| TEXAS INSTRUMENTS INCORPORATED
| Standard Linear and Logic Group
| IBIS Model of SN74LVCH16T245
| 16-Bit Dual-Supply Bus Transceiver With Configurable Voltage
| Translation and 3-State Outputs
| This file contains package information for the following:
|  TSSOP 48-pin (DGG) package as [Component] LVCH16T245_DGG
|  TVSOP 48-pin (DGV) package as [Component] LVCH16T245_DGV
|  VFBGA 48-pin (GQL) package as [Component] LVCH16T245_GQL
|  VFBGA 48-pin (ZQL) package as [Component] LVCH16T245_ZQL
| This device can be powered at the following Vccs:
|  1.8 volt Vcc
|  2.5 volt Vcc
|  3.3 volt Vcc
|  5 volt Vcc
| This file provides unique models under the [Model Selector] for each Vcc.
| For operation at a specific Vcc, select the appropriate model after each
| [Model Selector] keyword.
[IBIS Ver]   3.2
[Comment char]  |_char
[File Name]   sn74lvch16t245.ibs
[File Rev]   1.1 | x_die
[Date]   October 04, 2005
[Source]   Data created from TI-SPICE simulations at TI-SLL.
[Notes]   The following is an IBIS list for the LVCH16T245.
   Please contact sllibis@ti.com with questions and
   comments concerning SLL IBIS models.
   - FILE REV HISTORY
   - 1.1 Release IBIS file on 09/20/05
   - Power-clamp data has been deleted since there is no
   power-clamp diode in the device.
   - Due to presence of bus hold at input, GND-clamp curves
   have non-monotonic warnings.
   - Due to the fact that the Device is 5-V Input/Output
   tolarent, the output model has some Non-Monotonic Warnings.
[Disclaimer] Property of Texas Instruments Incorporated.  Unauthorized
   reproduction and/or distribution is strictly prohibited.
   This product is protected under copyright law.
   Created  2005, (C) Copyright  2005, Texas Instruments
   Incorporated, All Rights Reserved
   UNLESS THERE IS A SIGNED, WRITTEN AGREEMENT TO THE
   CONTRARY, TEXAS INSTRUMENTS (TI) IS PROVIDING THE IBIS
   MODELS  AND WITHOUT ANY WARRANTY, EXPRESSED OR
   IMPLIED.  TI assumes no liability for:
   1) the accuracy of the IBIS models provided to your
   company;
   2) the proper functioning of these IBIS Models in your
   design or for any resulting applications; or
   3) infringement of patents, copyrights or intellectual
   property rights resulting from your use of these IBIS
   models.
   TI provides IBIS Models as a service to our customers.
   You and your company shall not distribute, sell or give
   these models to anyone else without prior written
   permission from TI.
   TI reserves the right to make changes to our products or
   to discontinue any semiconductor product or service
   without notice, and advises our customers to obtain the
   latest version of relevant information to verify, before
   placing orders, that the information being relied on is
   current.
   Please be aware that your receipt and use of the IBIS
   information provided shall serve as acceptance of these
   terms and conditions.  If you do not accept these terms,
   you should return or destroy the IBIS models and any
   other accompanying information immediately.
| Component LVCH16T245_DGG 48-pin TSSOP
[Component]   LVCH16T245_DGG
[Manufacturer]   Texas Instruments, Inc.
[Package]
|   typ   min   max
R_pkg   4.400e-02   3.800e-02   5.100e-02
L_pkg   3.019e-09   2.486e-09   4.099e-09
C_pkg   5.070e-13   3.340e-13   8.090e-13
[Pin]   signal_name   model_name   R_pin   L_pin   C_pin
1   1DIR   LVCH16T245_DIR   4.100e-02   4.017e-09   7.590e-13
2   1B1   LVCH16T245_IO   4.200e-02   3.737e-09   7.920e-13
3   1B2   LVCH16T245_IO   4.200e-02   3.480e-09   6.610e-13
4   GND   GND   3.800e-02   3.131e-09   5.750e-13
5   1B3   LVCH16T245_IO   4.700e-02   3.122e-09   5.660e-13
6   1B4   LVCH16T245_IO   4.300e-02   2.948e-09   5.040e-13
7   VCCB   POWER   4.500e-02   2.845e-09   3.970e-13
8   1B5   LVCH16T245_IO   4.900e-02   2.835e-09   3.940e-13
9   1B6   LVCH16T245_IO   4.800e-02   2.715e-09   3.780e-13
10   GND   GND   5.000e-02   2.664e-09   3.630e-13
11   1B7   LVCH16T245_IO   5.000e-02   2.585e-09   3.480e-13
12   1B8   LVCH16T245_IO   4.900e-02   2.550e-09   3.370e-13
13   2B1   LVCH16T245_IO   4.900e-02   2.541e-09   3.360e-13
14   2B2   LVCH16T245_IO   5.000e-02   2.574e-09   3.480e-13
15   GND   GND   4.900e-02   2.618e-09   3.590e-13
16   2B3   LVCH16T245_IO   4.600e-02   2.671e-09   3.750e-13
17   2B4   LVCH16T245_IO   4.500e-02   2.754e-09   3.890e-13
18   VCCB   POWER   4.400e-02   2.823e-09   4.500e-13
19   2B5   LVCH16T245_IO   4.200e-02   2.968e-09   5.030e-13
20   2B6   LVCH16T245_IO   5.100e-02   3.108e-09   5.350e-13
21   GND   GND   4.200e-02   3.175e-09   5.870e-13
22   2B7   LVCH16T245_IO   4.100e-02   3.449e-09   6.780e-13
23   2B8   LVCH16T245_IO   4.400e-02   3.766e-09   8.040e-13
24   2DIR   LVCH16T245_DIR   4.300e-02   4.065e-09   7.610e-13
25   2NOE   LVCH16T245_NOE   4.100e-02   3.994e-09   7.570e-13
26   2A8   LVCH16T245_IO   3.900e-02   3.649e-09   7.890e-13
27   2A7   LVCH16T245_IO   3.800e-02   3.362e-09   6.600e-13
28   GND   GND   3.800e-02   3.082e-09   5.740e-13
29   2A6   LVCH16T245_IO   4.400e-02   2.990e-09   5.220e-13
30   2A5   LVCH16T245_IO   4.100e-02   2.917e-09   4.950e-13
31   VCCA   POWER   4.300e-02   2.820e-09   4.480e-13
32   2A4   LVCH16T245_IO   4.300e-02   2.699e-09   3.850e-13
33   2A3   LVCH16T245_IO   4.500e-02   2.628e-09   3.720e-13
34   GND   GND   4.600e-02   2.556e-09   3.560e-13
35   2A2   LVCH16T245_IO   4.600e-02   2.495e-09   3.440e-13
36   2A1   LVCH16T245_IO   4.700e-02   2.487e-09   3.340e-13
37   1A8   LVCH16T245_IO   4.700e-02   2.490e-09   3.350e-13
38   1A7   LVCH16T245_IO   4.600e-02   2.486e-09   3.430e-13
39   GND   GND   4.500e-02   2.566e-09   3.560e-13
40   1A6   LVCH16T245_IO   4.400e-02   2.639e-09   3.740e-13
41   1A5   LVCH16T245_IO   4.300e-02   2.701e-09   3.860e-13
42   VCCA   POWER   4.300e-02   2.817e-09   4.500e-13
43   1A4   LVCH16T245_IO   4.100e-02   2.935e-09   5.010e-13
44   1A3   LVCH16T245_IO   4.700e-02   3.035e-09   5.290e-13
45   GND   GND   4.300e-02   3.171e-09   5.890e-13
46   1A2   LVCH16T245_IO   4.000e-02   3.415e-09   6.820e-13
47   1A1   LVCH16T245_IO   4.300e-02   3.741e-09   8.090e-13
48   1NOE   LVCH16T245_NOE   4.400e-02   4.099e-09   7.640e-13
| Component LVCH16T245_DGV 48-pin TVSOP
[Component]   LVCH16T245_DGV
[Manufacturer]   Texas Instruments, Inc.
[Package]
|   typ   min   max
R_pkg   7.000e-02   4.900e-02   8.500e-02
L_pkg   3.013e-09   2.743e-09   3.408e-09
C_pkg   3.710e-13   2.940e-13   5.110e-13
[Pin]   signal_name   model_name   R_pin   L_pin   C_pin
1   1DIR   LVCH16T245_DIR   4.900e-02   3.393e-09   4.970e-13
2   1B1   LVCH16T245_IO   6.000e-02   3.250e-09   5.020e-13
3   1B2   LVCH16T245_IO   7.700e-02   3.310e-09   4.510e-13
4   GND   GND   8.500e-02   3.299e-09   4.040e-13
5   1B3   LVCH16T245_IO   8.300e-02   3.136e-09   3.600e-13
6   1B4   LVCH16T245_IO   7.700e-02   3.019e-09   3.630e-13
7   VCCB   POWER   6.500e-02   2.882e-09   3.490e-13
8   1B5   LVCH16T245_IO   6.600e-02   2.829e-09   3.140e-13
9   1B6   LVCH16T245_IO   6.700e-02   2.796e-09   3.140e-13
10   GND   GND   6.900e-02   2.754e-09   3.080e-13
11   1B7   LVCH16T245_IO   7.000e-02   2.753e-09   3.010e-13
12   1B8   LVCH16T245_IO   7.100e-02   2.745e-09   2.940e-13
13   2B1   LVCH16T245_IO   7.000e-02   2.744e-09   2.940e-13
14   2B2   LVCH16T245_IO   7.000e-02   2.754e-09   3.010e-13
15   GND   GND   6.900e-02   2.754e-09   3.080e-13
16   2B3   LVCH16T245_IO   6.700e-02   2.796e-09   3.140e-13
17   2B4   LVCH16T245_IO   6.600e-02   2.829e-09   3.140e-13
18   VCCB   POWER   6.500e-02   2.883e-09   3.500e-13
19   2B5   LVCH16T245_IO   7.500e-02   3.014e-09   3.630e-13
20   2B6   LVCH16T245_IO   8.000e-02   3.128e-09   3.580e-13
21   GND   GND   8.400e-02   3.295e-09   4.030e-13
22   2B7   LVCH16T245_IO   7.800e-02   3.311e-09   4.520e-13
23   2B8   LVCH16T245_IO   6.200e-02   3.259e-09   5.010e-13
24   2DIR   LVCH16T245_DIR   5.200e-02   3.404e-09   4.960e-13
25   2NOE   LVCH16T245_NOE   5.300e-02   3.397e-09   5.050e-13
26   2A8   LVCH16T245_IO   6.200e-02   3.249e-09   5.110e-13
27   2A7   LVCH16T245_IO   7.700e-02   3.308e-09   4.530e-13
28   GND   GND   8.200e-02   3.289e-09   4.030e-13
29   2A6   LVCH16T245_IO   7.800e-02   3.121e-09   3.590e-13
30   2A5   LVCH16T245_IO   7.400e-02   3.010e-09   3.630e-13
31   VCCA   POWER   6.500e-02   2.883e-09   3.490e-13
32   2A4   LVCH16T245_IO   6.700e-02   2.829e-09   3.140e-13
33   2A3   LVCH16T245_IO   6.700e-02   2.795e-09   3.140e-13
34   GND   GND   6.900e-02   2.753e-09   3.070e-13
35   2A2   LVCH16T245_IO   7.000e-02   2.753e-09   3.010e-13
36   2A1   LVCH16T245_IO   7.000e-02   2.743e-09   2.940e-13
37   1A8   LVCH16T245_IO   7.000e-02   2.743e-09   2.940e-13
38   1A7   LVCH16T245_IO   7.000e-02   2.753e-09   3.010e-13
39   GND   GND   6.900e-02   2.754e-09   3.070e-13
40   1A6   LVCH16T245_IO   6.800e-02   2.797e-09   3.140e-13
41   1A5   LVCH16T245_IO   6.700e-02   2.830e-09   3.140e-13
42   VCCA   POWER   6.400e-02   2.880e-09   3.490e-13
43   1A4   LVCH16T245_IO   7.200e-02   3.004e-09   3.620e-13
44   1A3   LVCH16T245_IO   7.800e-02   3.121e-09   3.590e-13
45   GND   GND   8.400e-02   3.296e-09   4.030e-13
46   1A2   LVCH16T245_IO   7.700e-02   3.308e-09   4.510e-13
47   1A1   LVCH16T245_IO   6.200e-02   3.258e-09   4.990e-13
48   1NOE   LVCH16T245_NOE   5.300e-02   3.408e-09   4.940e-13
| Component LVCH16T245_GQL 48-pin VFBGA
[Component]   LVCH16T245_GQL
[Manufacturer]   Texas Instruments, Inc.
[Package]
|   typ   min   max
R_pkg   7.900e-02   4.500e-02   9.400e-02
L_pkg   2.264e-09   1.398e-09   2.722e-09
C_pkg   3.060e-13   1.170e-13   4.040e-13
[Pin]   signal_name   model_name   R_pin   L_pin   C_pin
A1   1DIR   LVCH16T245_DIR   5.100e-02   1.531e-09   2.100e-13
B2   1B1   LVCH16T245_IO   7.300e-02   2.572e-09   3.120e-13
B1   1B2   LVCH16T245_IO   7.100e-02   1.835e-09   2.320e-13
B3   GND   GND   9.400e-02   2.717e-09   3.830e-13
C2   1B3   LVCH16T245_IO   8.900e-02   2.534e-09   3.500e-13
C1   1B4   LVCH16T245_IO   7.100e-02   1.831e-09   2.310e-13
C3   VCCB   POWER   9.400e-02   2.722e-09   3.920e-13
D2   1B5   LVCH16T245_IO   9.000e-02   2.551e-09   3.520e-13
D1   1B6   LVCH16T245_IO   7.200e-02   1.846e-09   2.440e-13
D3   GND   GND   9.400e-02   2.719e-09   4.030e-13
E2   1B7   LVCH16T245_IO   8.900e-02   2.541e-09   3.510e-13
E1   1B8   LVCH16T245_IO   7.200e-02   1.850e-09   2.270e-13
F1   2B1   LVCH16T245_IO   7.200e-02   1.850e-09   2.270e-13
F2   2B2   LVCH16T245_IO   8.900e-02   2.541e-09   3.510e-13
G3   GND   GND   9.400e-02   2.718e-09   4.040e-13
G1   2B3   LVCH16T245_IO   7.200e-02   1.847e-09   2.440e-13
G2   2B4   LVCH16T245_IO   9.000e-02   2.551e-09   3.520e-13
H3   VCCB   POWER   9.400e-02   2.721e-09   3.920e-13
H1   2B5   LVCH16T245_IO   7.000e-02   1.830e-09   2.310e-13
H2   2B6   LVCH16T245_IO   8.800e-02   2.524e-09   3.500e-13
J3   GND   GND   9.300e-02   2.709e-09   3.820e-13
J1   2B7   LVCH16T245_IO   7.100e-02   1.851e-09   2.330e-13
J2   2B8   LVCH16T245_IO   5.600e-02   2.605e-09   3.900e-13
K1   2DIR   LVCH16T245_DIR   4.500e-02   1.398e-09   1.170e-13
K6   2NOE   LVCH16T245_NOE   4.500e-02   1.512e-09   1.930e-13
J5   2A8   LVCH16T245_IO   5.500e-02   2.492e-09   3.130e-13
J6   2A7   LVCH16T245_IO   7.000e-02   1.821e-09   2.300e-13
J4   GND   GND   9.300e-02   2.703e-09   3.820e-13
H5   2A6   LVCH16T245_IO   8.900e-02   2.529e-09   3.500e-13
H6   2A5   LVCH16T245_IO   7.100e-02   1.826e-09   2.300e-13
H4   VCCA   POWER   9.400e-02   2.722e-09   3.910e-13
G5   2A4   LVCH16T245_IO   9.000e-02   2.551e-09   3.520e-13
G6   2A3   LVCH16T245_IO   7.200e-02   1.846e-09   2.440e-13
G4   GND   GND   9.400e-02   2.719e-09   4.040e-13
F5   2A2   LVCH16T245_IO   8.800e-02   2.510e-09   3.490e-13
F6   2A1   LVCH16T245_IO   7.200e-02   1.850e-09   2.270e-13
E6   1A8   LVCH16T245_IO   7.100e-02   1.850e-09   2.270e-13
E5   1A7   LVCH16T245_IO   8.900e-02   2.529e-09   3.500e-13
D4   GND   GND   9.400e-02   2.719e-09   4.030e-13
D6   1A6   LVCH16T245_IO   7.200e-02   1.847e-09   2.430e-13
D5   1A5   LVCH16T245_IO   8.900e-02   2.550e-09   3.520e-13
C4   VCCA   POWER   9.400e-02   2.722e-09   3.910e-13
C6   1A4   LVCH16T245_IO   7.100e-02   1.827e-09   2.300e-13
C5   1A3   LVCH16T245_IO   8.900e-02   2.539e-09   3.500e-13
B4   GND   GND   9.300e-02   2.705e-09   3.820e-13
B6   1A2   LVCH16T245_IO   7.100e-02   1.831e-09   2.270e-13
B5   1A1   LVCH16T245_IO   7.300e-02   2.685e-09   3.800e-13
A6   1NOE   LVCH16T245_NOE   5.100e-02   1.417e-09   1.330e-13
| Component LVCH16T245_ZQL 48-pin VFBGA
[Component]   LVCH16T245_ZQL
[Manufacturer]   Texas Instruments, Inc.
[Package]
|   typ   min   max
R_pkg   7.900e-02   4.500e-02   9.400e-02
L_pkg   2.264e-09   1.398e-09   2.722e-09
C_pkg   3.060e-13   1.170e-13   4.040e-13
[Pin]   signal_name   model_name   R_pin   L_pin   C_pin
A1   1DIR   LVCH16T245_DIR   5.100e-02   1.531e-09   2.100e-13
B2   1B1   LVCH16T245_IO   7.300e-02   2.572e-09   3.120e-13
B1   1B2   LVCH16T245_IO   7.100e-02   1.835e-09   2.320e-13
B3   GND   GND   9.400e-02   2.717e-09   3.830e-13
C2   1B3   LVCH16T245_IO   8.900e-02   2.534e-09   3.500e-13
C1   1B4   LVCH16T245_IO   7.100e-02   1.831e-09   2.310e-13
C3   VCCB   POWER   9.400e-02   2.722e-09   3.920e-13
D2   1B5   LVCH16T245_IO   9.000e-02   2.551e-09   3.520e-13
D1   1B6   LVCH16T245_IO   7.200e-02   1.846e-09   2.440e-13
D3   GND   GND   9.400e-02   2.719e-09   4.030e-13
E2   1B7   LVCH16T245_IO   8.900e-02   2.541e-09   3.510e-13
E1   1B8   LVCH16T245_IO   7.200e-02   1.850e-09   2.270e-13
F1   2B1   LVCH16T245_IO   7.200e-02   1.850e-09   2.270e-13
F2   2B2   LVCH16T245_IO   8.900e-02   2.541e-09   3.510e-13
G3   GND   GND   9.400e-02   2.718e-09   4.040e-13
G1   2B3   LVCH16T245_IO   7.200e-02   1.847e-09   2.440e-13
G2   2B4   LVCH16T245_IO   9.000e-02   2.551e-09   3.520e-13
H3   VCCB   POWER   9.400e-02   2.721e-09   3.920e-13
H1   2B5   LVCH16T245_IO   7.000e-02   1.830e-09   2.310e-13
H2   2B6   LVCH16T245_IO   8.800e-02   2.524e-09   3.500e-13
J3   GND   GND   9.300e-02   2.709e-09   3.820e-13
J1   2B7   LVCH16T245_IO   7.100e-02   1.851e-09   2.330e-13
J2   2B8   LVCH16T245_IO   5.600e-02   2.605e-09   3.900e-13
K1   2DIR   LVCH16T245_DIR   4.500e-02   1.398e-09   1.170e-13
K6   2NOE   LVCH16T245_NOE   4.500e-02   1.512e-09   1.930e-13
J5   2A8   LVCH16T245_IO   5.500e-02   2.492e-09   3.130e-13
J6   2A7   LVCH16T245_IO   7.000e-02   1.821e-09   2.300e-13
J4   GND   GND   9.300e-02   2.703e-09   3.820e-13
H5   2A6   LVCH16T245_IO   8.900e-02   2.529e-09   3.500e-13
H6   2A5   LVCH16T245_IO   7.100e-02   1.826e-09   2.300e-13
H4   VCCA   POWER   9.400e-02   2.722e-09   3.910e-13
G5   2A4   LVCH16T245_IO   9.000e-02   2.551e-09   3.520e-13
G6   2A3   LVCH16T245_IO   7.200e-02   1.846e-09   2.440e-13
G4   GND   GND   9.400e-02   2.719e-09   4.040e-13
F5   2A2   LVCH16T245_IO   8.800e-02   2.510e-09   3.490e-13
F6   2A1   LVCH16T245_IO   7.200e-02   1.850e-09   2.270e-13
E6   1A8   LVCH16T245_IO   7.100e-02   1.850e-09   2.270e-13
E5   1A7   LVCH16T245_IO   8.900e-02   2.529e-09   3.500e-13
D4   GND   GND   9.400e-02   2.719e-09   4.030e-13
D6   1A6   LVCH16T245_IO   7.200e-02   1.847e-09   2.430e-13
D5   1A5   LVCH16T245_IO   8.900e-02   2.550e-09   3.520e-13
C4   VCCA   POWER   9.400e-02   2.722e-09   3.910e-13
C6   1A4   LVCH16T245_IO   7.100e-02   1.827e-09   2.300e-13
C5   1A3   LVCH16T245_IO   8.900e-02   2.539e-09   3.500e-13
B4   GND   GND   9.300e-02   2.705e-09   3.820e-13
B6   1A2   LVCH16T245_IO   7.100e-02   1.831e-09   2.270e-13
B5   1A1   LVCH16T245_IO   7.300e-02   2.685e-09   3.800e-13
A6   1NOE   LVCH16T245_NOE   5.100e-02   1.417e-09   1.330e-13
| Model LVCH16T245_NOE
[Model Selector]   LVCH16T245_NOE
LVCH16T245_NOE_18   1.8 volt Vcc
LVCH16T245_NOE_25   2.5 volt Vcc
LVCH16T245_NOE_33   3.3 volt Vcc
LVCH16T245_NOE_50   5 volt Vcc
| Model LVCH16T245_DIR
[Model Selector]   LVCH16T245_DIR
LVCH16T245_DIR_18   1.8 volt Vcc
LVCH16T245_DIR_25   2.5 volt Vcc
LVCH16T245_DIR_33   3.3 volt Vcc
LVCH16T245_DIR_50   5 volt Vcc
| Model LVCH16T245_IO
[Model Selector]   LVCH16T245_IO
LVCH16T245_IO_18   1.8 volt Vcc
LVCH16T245_IO_25   2.5 volt Vcc
LVCH16T245_IO_33   3.3 volt Vcc
LVCH16T245_IO_50   5 volt Vcc
| Models and submodels in the file (12): LVCH16T245_NOE_18 (Input), LVCH16T245_NOE_25 (Input), LVCH16T245_NOE_33 (Input), LVCH16T245_NOE_50 (Input), LVCH16T245_DIR_18 (Input), LVCH16T245_DIR_25 (Input), LVCH16T245_DIR_33 (Input), LVCH16T245_DIR_50 (Input), LVCH16T245_IO_18 (I/O), LVCH16T245_IO_25 (I/O), LVCH16T245_IO_33 (I/O), LVCH16T245_IO_50 (I/O)
